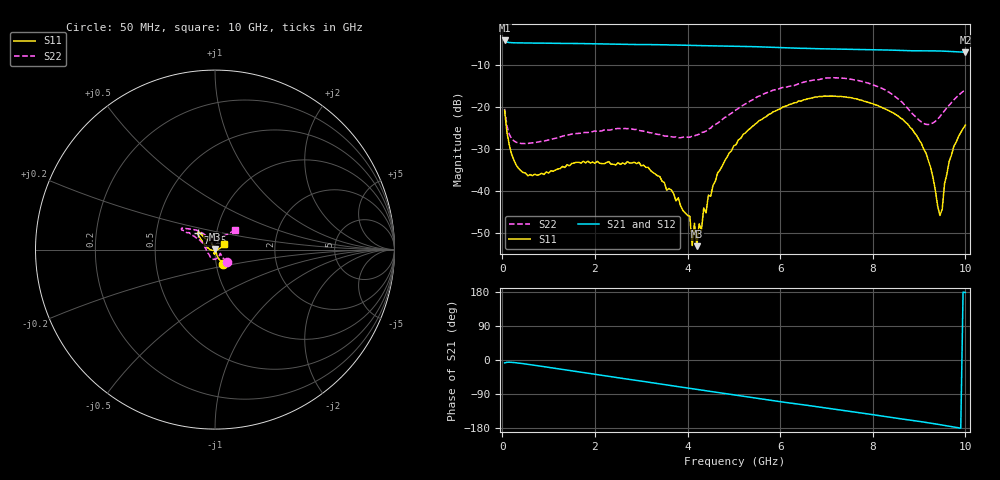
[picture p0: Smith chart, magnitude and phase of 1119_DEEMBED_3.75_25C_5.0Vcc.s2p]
!Hittite Microwave Corp.
!Digital Attenuator/PhaseShifter Rev 1.4.0
!Filename: C:\DATA\DATA\1119_DEEMBED_3.75_25C_5.0Vcc.s2p
!VNA ID: Agilent Technologies,N5224A,MY51441122,A.10.45.03
!Device type:
!2 Port Calibration.
!Temp(C): 25
!Lot Number:
!Serial Number:
!Operator:
!Misc:
!Attenuator:  3.750
# GHZ S DB R 50.0
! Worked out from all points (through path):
!   200 points, 50 MHz to 10 GHz, reference 50 ohm
!   highest |S21| = -4.23 dB at 50 MHz (marker M1); lowest = -7.0 dB at 10 GHz (marker M2)
!   group delay of S21, straight-line fit = 49.5 ps
!   lowest |S11| = -53.2 dB at 4.2 GHz (marker M3), VSWR 1.00, Z = 50.2 + j0.131 ohm
!   |S11| at or under -10 dB: start of sweep to end of sweep
!   |S22| runs from -28.8 to -13.1 dB; largest |S21 - S12| = 0.0019
!   S11 on the Smith chart (normalised r, x): 50 MHz: 1.08, -0.17; 7.15 GHz: 0.81, +0.16; 10 GHz: 1.10, +0.07
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0.05  -20.87 -61.0  -4.23 -7.7  -4.23 -7.7  -20.52 -46.8
0.2  -31.27 -71.1  -4.76 -6.1  -4.76 -6.1  -27.59 -38.9
0.55  -36.46 -69.7  -4.84 -11.3  -4.83 -11.3  -28.76 -37.4
1.75  -33.01 -101.9  -4.98 -33.1  -4.98 -33.2  -26.18 -73.6
3.4  -36.61 -91.8  -5.25 -63.0  -5.25 -63.0  -26.64 -128.3
4.05  -46.11 -47.9  -5.39 -74.8  -5.40 -74.8  -27.27 -161.8
4.1  -53.06 -9.2  -5.40 -75.8  -5.41 -75.8  -27.03 -165.2
4.15  -47.75 -8.4  -5.42 -76.7  -5.43 -76.7  -26.92 -169.1
4.2  -53.21 36.8  -5.44 -77.5  -5.45 -77.6  -26.74 -173.1
4.25  -47.90 33.6  -5.45 -78.4  -5.46 -78.5  -26.55 -175.3
4.3  -49.41 78.7  -5.46 -79.3  -5.47 -79.4  -26.15 -180.0
4.35  -44.13 70.3  -5.47 -80.1  -5.48 -80.2  -26.05 176.2
4.45  -41.06 90.3  -5.49 -82.0  -5.51 -82.1  -25.32 171.1
5.05  -29.01 120.3  -5.60 -92.7  -5.62 -92.8  -20.75 149.0
6.7  -17.88 132.7  -6.15 -121.6  -6.16 -121.6  -13.70 148.9
7.15  -17.51 135.1  -6.25 -129.2  -6.27 -129.2  -13.10 147.7
8.35  -20.96 145.3  -6.52 -150.6  -6.52 -150.6  -16.55 133.5
9.05  -28.75 170.8  -6.69 -162.9  -6.70 -162.9  -23.62 112.8
9.25  -34.47 -169.5  -6.70 -166.6  -6.72 -166.7  -24.11 92.1
9.45  -45.90 -68.5  -6.74 -170.7  -6.76 -170.7  -22.36 67.3
9.65  -33.03 10.0  -6.84 -174.8  -6.85 -174.8  -19.63 52.2
10  -24.37 33.7  -7.04 178.0  -7.05 178.1  -16.01 44.6
